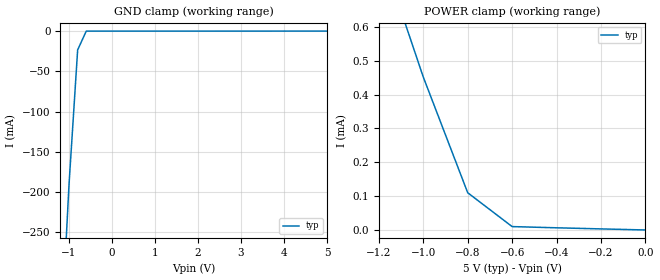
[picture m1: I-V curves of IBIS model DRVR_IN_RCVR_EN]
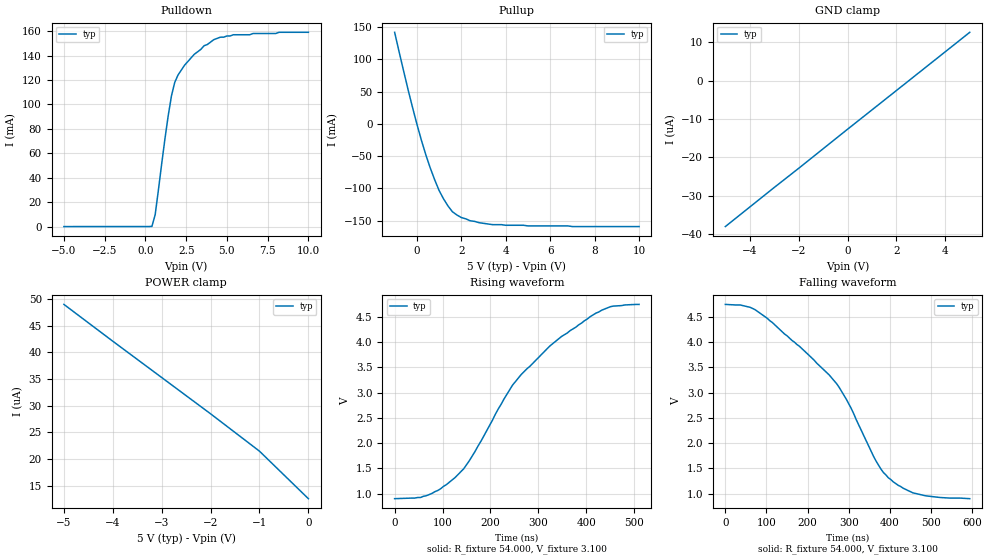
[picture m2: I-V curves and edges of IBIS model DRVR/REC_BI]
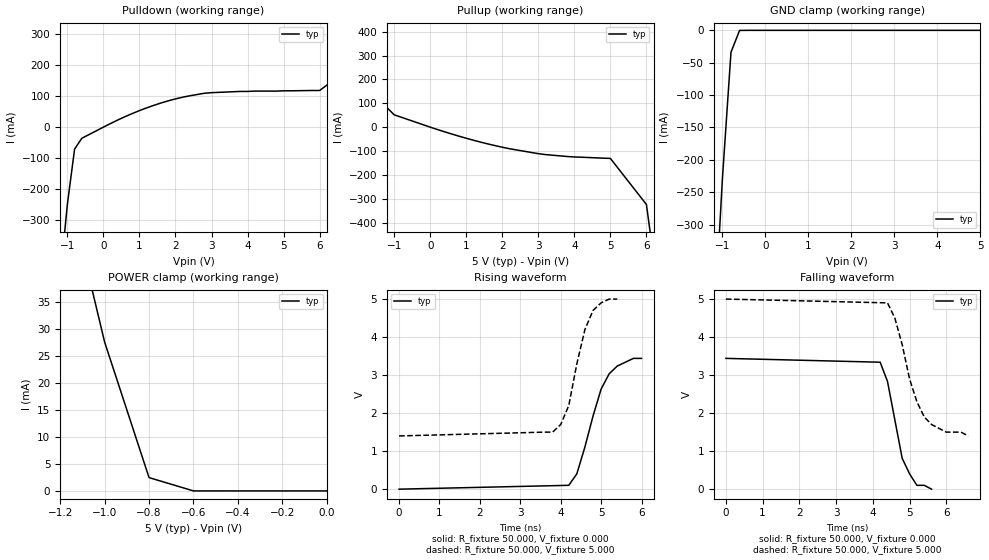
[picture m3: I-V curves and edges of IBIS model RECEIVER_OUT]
|   Texas Instruments Incorporated
|   Data Transmissions Products
|   IBIS Model for SN65HVD07
|   8D SOIC Package
[IBIS Ver]   3.2
[Comment char]   |_char
[File name]   hvd07.ibs
[File Rev]   1.1
[Date]   11Apr07
[Source]   File originated at Texas Instruments Incorporated.
   Data Transmission Products Group.
[Notes]
[Disclaimer]
(C) Copyright Texas Instruments Incorporated 2002
   All rights reserved
  Texas Instruments Incorporated hereby grants 1the user of this IBIS
model a non-exclusive, nontransferable license to use this IBIS model
under the following terms.  Before using this IBIS model, the user
should read this license.  If the user does not accept these terms,
the IBIS model should be returned to Texas Instruments within 30 days.
  The user is granted this license only to use the IBIS model and
is not granted rights to sell, load, rent, lease or license the IBIS
model in whole or in part, or in modified form to anyone other than
user.  User may modify the IBIS model to suit its specific applications
but rights to derivative works and such modifications shall belong to
Texas Instruments.
  This IBIS model is provided on an "AS IS" basis and Texas Instruments
makes absolutely no warranty with respect to the information contained
herein.  TEXAS INSTRUMENTS DISCLAIMS AND CUSTOMER WAIVES ALL WARRANTIES,
EXPRESS OR IMPLIED, INCLUDING WARRANTIES OF MERCHANTABILITY OR FITNESS
FOR A PARTICULAR PURPOSE. The entire risk as to quality and performance
is with the Customer. ACCORDINGLY, IN NO EVENT SHALL THE COMPANY BE LIABLE
FOR ANY DAMAGES, WHETHER IN CONTRACT OR TORT,INCLUDING ANY LOST PROFITS
OR OTHER INCIDENTAL, CONSEQUENTIAL, EXEMPLARY, OR PUNITIVE DAMAGES ARISING
OUT OF THE USE OR APPLICATION OF THE IBIS model provided in this package.
Further, Texas Instruments reserves the right to discontinue or make changes
without notice to any product herein to improve reliability, function, or
design. Texas Instruments does not convey any license under patent rights
or any other intellectual property rights, including those of third parties.
Contact Texas Instruments at ATTN:DATA TRANSMISSIONS
[Copyright]   Copyright 2002, Texas Instruments, All Rights Reserved
[Component]   HVD07D
[Manufacturer]  Texas Instruments Incorporated
[Package]
|   typ   min   max
R_pkg   0.036   0.033   0.039
L_pkg   3.340nH   2.445nH   4.233nH
C_pkg   0.470pF   0.308pF   0.631pF
[Pin]   signal_name   model_name   R_pin   L_pin   C_pin
1   R   RECEIVER_OUT   0.034   4.233n   0.630p
2   RE   DRVR_IN_RCVR_EN   0.038   2.445n   0.309p
3   DE   DRIVER_EN   0.039   2.448n   0.309p
4   D   DRVR_IN_RCVR_EN   0.033   4.231n   0.631p
5   GND   GND   0.033   4.230n   0.630p
6   A   DRVR/REC_BI   0.039   2.450n   0.308p
7   B   DRVR/REC_BI   0.039   2.448n   0.309p
8   VCC   POWER   0.033   4.231n   0.630p
[Diff_pin]   inv_pin   vdiff   tdelay_typ   tdelay_min   tdelay_max
| The 'A' pin is Diff_pin and the 'B' pin is the inv_pin
6   7   0.200   0 0 0
| Models and submodels in the file (4): DRVR_IN_RCVR_EN (Input), DRIVER_EN (Input), DRVR/REC_BI (I/O), RECEIVER_OUT (3-state)
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|   Driver Input / Receiver Enable Model
[Model]   DRVR_IN_RCVR_EN
Model_type   Input
|Signals   D,RE
Vinh = 2.0
Vinl = 0.8
|   typ   min   max
C_comp   1.0pF   NA   NA
|   typ   min   max
[Temperature Range]   25.0   NA   NA
[Voltage range]   5.0V   4.5V   5.5V
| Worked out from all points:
|   GND clamp passes 1 mA (typ) near -0.61 V on its own axis
|   POWER clamp passes 1 mA (typ) near -1.28 V on its own axis
[GND_clamp]
|   Voltage   I(typ)   I(min)   I(max)
-5V       -4.2A      NA         NA
-4V       -3.22A     NA         NA
-3V       -2.23A     NA         NA
-2V       -1.22A     NA         NA
-1V       -190mA     NA         NA
-800mV    -23.4mA    NA         NA
-600mV    -55.7uA    NA         NA
-400mV    -27.7uA    NA         NA
-200mV    -27.7uA    NA         NA
0V        -27.6uA    NA         NA
2.4V      -25.3uA    NA         NA
5V        12pA       NA         NA
[Power_clamp]
| Note that the[POWER_clamp]voltage table is referenced to Vcc
| and is calculated using Vtable=Vcc - Vmeasured.
|   Voltage   I(typ)   I(min)   I(max)
-5V       8.78mA     NA         NA
-1.2V     841uA      NA         NA
-1V       452uA      NA         NA
-800mV    110uA      NA         NA
-600mV    10uA       NA         NA
0V        12pA       NA         NA
|   Driver Output / Receiver Input Model
[Model]   DRVR/REC_BI
Model_type   I/O
| Signals   A,B
Vinl = 4.3V
Vinh = 1.0V
Vmeas = 3.1V   |Reference voltage for timing measurements
Cref = 50pF   |Timing specification test load capacitance value
Rref = 54   |Note: 54 Ohm load; single ended configuration
|   Timing specification test load voltage
| variable   typ   min   max
C_comp   32pF   26pF   38pF
|   typ   min   max
[Temperature Range]   25.0   NA   NA
[Voltage range]   5.0V   4.5V   5.5V
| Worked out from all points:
|   slope of the pulldown table from 0 to 0.75 V, typ, clamps not added: 30 ohm
|   slope of the pullup table from 0 to 0.75 V, typ, clamps not added: 9.18 ohm
|   rising waveform, R_fixture 54.000, V_fixture 3.100: 20-80 % time 174ns typ, NA min, NA max; typ from 0.9 V to 4.75 V
|   falling waveform, R_fixture 54.000, V_fixture 3.100: 20-80 % time 194ns typ, NA min, NA max; typ from 4.75 V to 0.9 V
[Pulldown]
|   Voltage   I(typ)   I(min)   I(max)
-5V       -38.1uA    NA         NA
400mV     107uA      NA         NA
600mV     9.71mA     NA         NA
1.2V      71.9mA     NA         NA
1.4V      90.8mA     NA         NA
1.6V      107mA      NA         NA
1.8V      118mA      NA         NA
2.4V      132mA      NA         NA
3.6V      148mA      NA         NA
4.6V      155mA      NA         NA
6.6V      158mA      NA         NA
10V       159mA      NA         NA
[Pullup]
|   Voltage   I(typ)   I(min)   I(max)
| Note that the[Pullup]voltage table is referenced to Vcc
| and is calculated using Vtable=Vcc - Vmeasured.
-1V       142mA      NA         NA
-200mV    26.4mA     NA         NA
200mV     -24.7mA    NA         NA
400mV     -47.4mA    NA         NA
600mV     -67.9mA    NA         NA
1V        -103mA     NA         NA
1.2V      -116mA     NA         NA
1.6V      -136mA     NA         NA
2V        -145mA     NA         NA
2.4V      -150mA     NA         NA
3.4V      -156mA     NA         NA
10V       -159mA     NA         NA
[GND_clamp]
|   Voltage   I(typ)   I(min)   I(max)
| Outputs in High Impedance (off)
-5V       -38.1uA    NA         NA
-4V       -33uA      NA         NA
-3V       -27.9uA    NA         NA
-2V       -22.9uA    NA         NA
-1V       -17.8uA    NA         NA
0V        -12.7uA    NA         NA
2.4V      -569nA     NA         NA
5V        12.6uA     NA         NA
[POWER_clamp]
|   Voltage   I(typ)   I(min)   I(max)
| Note that the [POWER_clamp] voltage table is referenced to Vcc
| and is calculated using Vtable = Vcc - Vmeasured.
| Outputs in Tri-state.
-5V       49uA       NA         NA
-4V       42.1uA     NA         NA
-3V       35.3uA     NA         NA
-2V       28.5uA     NA         NA
-1V       21.5uA     NA         NA
0V        12.6uA     NA         NA
[Ramp]
|   typ   min   max
dV/dt_r   2.00/174ns   NA   NA
dV/dt_f   2.00/192ns   NA   NA
R_load = 54ohm | Note: The measurement is on a differential configuration
|   with 54ohm line-to-line and a 10pF cap from each
|   line-to-ground.
[Rising Waveform]
R_fixture = 54.000
V_fixture = 3.100
C_fixture = 0.000
L_fixture = 0.000
|  time   V(typ)   V(min)   V(max)
0s        900.2mV    NA         NA
66ns      958.1mV    NA         NA
126ns     1.317V     NA         NA
156ns     1.654V     NA         NA
246ns     3.149V     NA         NA
276ns     3.473V     NA         NA
348ns     4.111V     NA         NA
432ns     4.633V     NA         NA
456ns     4.714V     NA         NA
510ns     4.748V     NA         NA
[Falling Waveform]
R_fixture = 54.000
V_fixture = 3.100
C_fixture = 0.000
L_fixture = 0.000
|  time   V(typ)   V(min)   V(max)
0s        4.748V     NA         NA
72ns      4.645V     NA         NA
252ns     3.354V     NA         NA
294ns     2.87V      NA         NA
366ns     1.649V     NA         NA
384ns     1.419V     NA         NA
408ns     1.234V     NA         NA
456ns     1.015V     NA         NA
486ns     957.8mV    NA         NA
594ns     900.2mV    NA         NA
[Model]   RECEIVER_OUT
Model_type   3-state
| Signals   R
Vmeas = 1.5V   |Reference voltage for timing measurements
Cref = 15pF   |Timing specification test load capacitance value
Vref = 0   |Timing specification test load voltage; GND
| variable   typ   min   max
C_comp   1.0pF   NA   NA
|   typ   min   max
[Temperature Range]   25.0   NA   NA
[Voltage range]   5.0V   4.5V   5.5V
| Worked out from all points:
|   slope of the pulldown table from 0 to 0.75 V, typ, clamps not added: 18.2 ohm
|   slope of the pullup table from 0 to 0.75 V, typ, clamps not added: 21 ohm
|   GND clamp passes 1 mA (typ) near -0.61 V on its own axis
|   POWER clamp passes 1 mA (typ) near -0.68 V on its own axis
|   rising waveform, R_fixture 50.000, V_fixture 0.000: 20-80 % time 580ps typ, NA min, NA max; typ from 0 V to 3.44 V
|   falling waveform, R_fixture 50.000, V_fixture 0.000: 20-80 % time 444ps typ, NA min, NA max; typ from 3.44 V to 0 V
|   rising waveform, R_fixture 50.000, V_fixture 5.000: 20-80 % time 464ps typ, NA min, NA max; typ from 1.4 V to 5 V
|   falling waveform, R_fixture 50.000, V_fixture 5.000: 20-80 % time 627ps typ, NA min, NA max; typ from 5 V to 1.4 V
[Pulldown]
|   Voltage   I(typ)   I(min)   I(max)
-5V       -4.95A     NA         NA
-2V       -1.44A     NA         NA
-1V       -249mA     NA         NA
-800mV    -70.9mA    NA         NA
-600mV    -35.9mA    NA         NA
400mV     23mA       NA         NA
1.6V      77.8mA     NA         NA
2.8V      109mA      NA         NA
6V        118mA      NA         NA
7V        204mA      NA         NA
8V        381mA      NA         NA
10V       741mA      NA         NA
[Pullup]
|   Voltage   I(typ)   I(min)   I(max)
| Note that the[Pullup]voltage table is referenced to Vcc
| and is calculated using Vtable=Vcc - Vmeasured.
-5V       741mA      NA         NA
-4V       560mA      NA         NA
-3V       380mA      NA         NA
-2V       202mA      NA         NA
-1V       51.7mA     NA         NA
800mV     -37.9mA    NA         NA
2.2V      -90.4mA    NA         NA
3.2V      -115mA     NA         NA
5V        -131mA     NA         NA
6V        -324mA     NA         NA
7V        -1.44A     NA         NA
10V       -4.95A     NA         NA
[GND_clamp]
|   Voltage   I(typ)   I(min)   I(max)
| Outputs in High Impedance (off)
-5V       -4.95A     NA         NA
-4V       -3.79A     NA         NA
-3V       -2.62A     NA         NA
-2V       -1.43A     NA         NA
-1V       -230mA     NA         NA
-800mV    -33.8mA    NA         NA
-600mV    -137uA     NA         NA
-400mV    -384nA     NA         NA
-200mV    -485pA     NA         NA
0V        -60pA      NA         NA
2V        -9.43pA    NA         NA
5V        66.4pA     NA         NA
[POWER_clamp]
|   Voltage   I(typ)   I(min)   I(max)
| Note that the [POWER_clamp] voltage table is referenced to Vcc
| and is calculated using Vtable = Vcc - Vmeasured.
| Outputs in Tri-state.
-5V       741mA      NA         NA
-4V       560mA      NA         NA
-3V       380mA      NA         NA
-2V       200mA      NA         NA
-1V       27.6mA     NA         NA
-800mV    2.47mA     NA         NA
-600mV    1.82uA     NA         NA
-400mV    894pA      NA         NA
-200mV    71.9pA     NA         NA
0V        66.4pA     NA         NA
[Ramp]
|   typ   min   max
dV/dt_r   4.10V/2.16ns   NA   NA
dV/dt_f   3.86V/3.15ns   NA   NA
R_load = 50
[Rising Waveform]
R_fixture = 50.000
V_fixture = 0.000
C_fixture = 0.000
L_fixture = 0.000
|  time   V(typ)   V(min)   V(max)
0s        2.127nV    NA         NA
4.2ns     101.2mV    NA         NA
4.4ns     404.7mV    NA         NA
4.6ns     1.113V     NA         NA
4.8ns     1.922V     NA         NA
5ns       2.631V     NA         NA
5.2ns     3.035V     NA         NA
5.4ns     3.238V     NA         NA
5.8ns     3.44V      NA         NA
6ns       3.44V      NA         NA
[Falling Waveform]
R_fixture = 50.000
V_fixture = 0.000
C_fixture = 0.000
L_fixture = 0.000
|  time   V(typ)   V(min)   V(max)
0s        3.44V      NA         NA
4.2ns     3.339V     NA         NA
4.4ns     2.833V     NA         NA
4.6ns     1.821V     NA         NA
4.8ns     809.4mV    NA         NA
5ns       404.7mV    NA         NA
5.2ns     101.2mV    NA         NA
5.4ns     101.2mV    NA         NA
5.6ns     2.127nV    NA         NA
[Rising Waveform]
R_fixture = 50.000
V_fixture = 5.000
C_fixture = 0.000
L_fixture = 0.000
|  time   V(typ)   V(min)   V(max)
0s        1.4V       NA         NA
3.8ns     1.5V       NA         NA
4ns       1.7V       NA         NA
4.2ns     2.2V       NA         NA
4.4ns     3.3V       NA         NA
4.6ns     4.2V       NA         NA
4.8ns     4.7V       NA         NA
5ns       4.9V       NA         NA
5.2ns     5V         NA         NA
5.4ns     5V         NA         NA
[Falling Waveform]
R_fixture = 50.000
V_fixture = 5.000
C_fixture = 0.000
L_fixture = 0.000
|  time   V(typ)   V(min)   V(max)
0s        5V         NA         NA
4.4ns     4.9V       NA         NA
4.6ns     4.5V       NA         NA
4.8ns     3.8V       NA         NA
5ns       2.9V       NA         NA
5.2ns     2.3V       NA         NA
5.4ns     1.9V       NA         NA
5.6ns     1.7V       NA         NA
6ns       1.5V       NA         NA
6.6ns     1.4V       NA         NA
